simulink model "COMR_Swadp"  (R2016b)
settings: Solver=FixedStepDiscrete  StartTime=0.0  StopTime=10.0  FixedStep=0.02  RelTol=1e-3  EnableMultiTasking=on
undefined symbols (not defined in the file or in its folder): bin2dec, COMR_ahBattNrmCap_C, COMR_cntNvmReadErr_CW, COMR_ti638LinComErr_C, COMR_tiNvmReadErr_C
libraries: simulink x93, dspswit3 x2
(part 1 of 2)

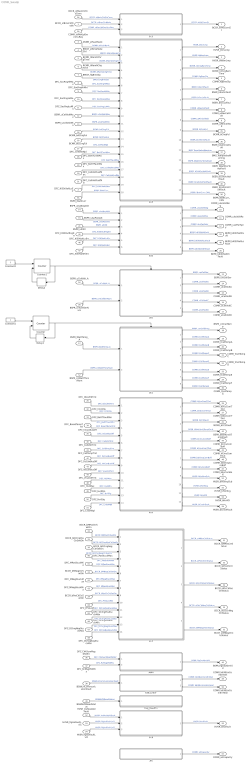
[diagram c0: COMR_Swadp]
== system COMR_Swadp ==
  BCCR_stBmsCtrMode : Inport
  DFC_Kl30cVoltLoErr : Inport  Port=2
  DSMR_stFaultRank : Inport  Port=3
  BMCR_stBmsModeCtrl : Inport  Port=4
  BCMR_tiRemDChrgTime : Inport  Port=5
  BCMR_tiRemAChgTime : Inport  Port=6
  BMCR_flgBmsSlp : Inport  Port=7
  DFC_SocRngHiMax : Inport  Port=8
  DFC_SocRngHiMin : Inport  Port=9
  DFC_SocRngLoMax : Inport  Port=10
  DFC_SocRngLoMin : Inport  Port=11
  BSPR_uCellVoltMax : Inport  Port=12
  BSPR_uCellVoltMin : Inport  Port=13
  BSPR_uIsoNegVolt : Inport  Port=14
  BSPR_uIsoPosVolt : Inport  Port=15
  BSPR_uCellVolt_A : Inport  Port=16
  BSPR_tBattTemp_A : Inport  Port=17
  BCMR_bAChrgFul : Inport  Port=18
  BCMR_bDChrgFul : Inport  Port=19
  DFC_Obc2E0Tmt : Inport  Port=20
  BSPR_uKl30 : Inport  Port=21
  BCCR_bMPosCtrSwtOn : Inport  Port=22
  BCCR_bMNegCtrSwtOn : Inport  Port=23
  BCCR_bPreChCtrSwtOn : Inport  Port=24
  BCCR_bDChrgPosCtrSwtOn : Inport  Port=25
  BCCR_bDChrgNegCtrSwtOn : Inport  Port=26
  DFC_CellVoltNpl : Inport  Port=27
  DFC_BattTCnstMax : Inport  Port=28
  DFC_BattTFaultMax : Inport  Port=29
  DFC_CellVoltFusfMax : Inport  Port=30
  DFC_CellVoltFusfMin : Inport  Port=31
  DFC_CC2Chk : Inport  Port=32
  DFC_BattTFaultMin : Inport  Port=33
  DFC_BoardTempTmt : Inport  Port=34
  DFC_InCanBusOff : Inport  Port=35
  DFC_ChkSumMsg050Err : Inport  Port=36
  DFC_RcMsg050Mis : Inport  Port=37
  BSWLinCommunicationFault : Inport  Port=38
  BSWNVMReadStatus : Inport  Port=39
  DFC_CellVoltTmt : Inport  Port=40
  DFC_CellTempTmt : Inport  Port=41
  DFC_DcCanBusOff : Inport  Port=42
  DFC_VeCanBusOff : Inport  Port=43
  DFC_Vcu2A3Tmt : Inport  Port=44
  DFC_Kl30OutRngErr : Inport  Port=45
  DFC_Kl30VoltLoErr : Inport  Port=46
  DFC_Kl30VoltHiErr : Inport  Port=47
  DFC_HvilMax : Inport  Port=48
  DFC_HvilMin : Inport  Port=49
  DFC_HvilSig : Inport  Port=50
  DFC_CrashNpl : Inport  Port=51
  HVSR_InsResValdFault : Inport  Port=52
  HVSR_flgIsoFaultLvl1 : Inport  Port=53
  HVSR_flgIsoFaultLvl2 : Inport  Port=54
  BSPR_iBattCurr : Inport  Port=55
  BCCR_stMainCtrDisConn : Inport  Port=56
  BSPR_cntBattTSnsrNum : Inport  Port=57
  BSPR_cntCellSerNum : Inport  Port=58
  COMR_stPwrUpDwnVcuReq : Inport  Port=59
  DFC_PosStuckMax : Inport  Port=60
  DFC_MPosStuckMin : Inport  Port=61
  DFC_MNegStuckMax : Inport  Port=62
  DFC_MNegStuckMin : Inport  Port=63
  DFC_PrStuckMin : Inport  Port=64
  DFC_DChrgPosStuckMax : Inport  Port=65
  DFC_DChrgPosStuckMin : Inport  Port=66
  DFC_DChrgNegStuckMax : Inport  Port=67
  DFC_DChrgNegStuckMin : Inport  Port=68
  2C2 : Subsystem
  2C8 : Subsystem
  2CE : Subsystem
  2CF : Subsystem
  3E0 : Subsystem
  3E1 : Subsystem
  615 : Subsystem
  616 : Subsystem
  638_LinErr : Subsystem
  ABM : Subsystem
  Ah : Subsystem
  Constant1 : Constant
  Constant2 : Constant
  Counter : dspswit3/Counter  Direction=Up  CountEvent=Non-zero sample  CounterSize=User defined  MaxCount=255  InitialCount=0  Output=Hit  HitValue=10  ResetInput=on  SamplesPerFrame=1  Ts=1  CntDtype=double  HitDtype=Logical
  Counter1 : dspswit3/Counter  Direction=Up  CountEvent=Non-zero sample  CounterSize=User defined  MaxCount=255  InitialCount=0  Output=Hit  HitValue=2  ResetInput=on  SamplesPerFrame=1  Ts=1  CntDtype=double  HitDtype=Logical
  Delay1 : Delay  DelayLength=1  InitialCondition=0
  Delay2 : Delay  DelayLength=1  InitialCondition=0
  Eep_ReadErr : Subsystem
  BCCR_stHVConnSt : Outport
  HVSR_bSrvLmp : Outport  Port=2
  HVSR_bWarnLmp : Outport  Port=3
  BCMR_tiChrgRemTime : Outport  Port=4
  COMR_flgBmsSlp : Outport  Port=5
  BSER_bSocHiFault : Outport  Port=6
  BSER_bSocLoFault : Outport  Port=7
  COMR_uMaxCellVolt : Outport  Port=8
  COMR_uMinCellVolt : Outport  Port=9
  COMR_uIsoVoltNeg : Outport  Port=10
  COMR_uIsoVoltPos : Outport  Port=11
  COMR_uLoPwrSply : Outport  Port=12
  BSPR_cntCellSer : Outport  Port=13
  COMR_uCellVoltA : Outport  Port=14
  COMR_uCellVoltB : Outport  Port=15
  COMR_uCellVoltC : Outport  Port=16
  COMR_uCellVoltD : Outport  Port=17
  BSPR_cntCellTemp : Outport  Port=18
  COMR_tCellTempA : Outport  Port=19
  COMR_tCellTempB : Outport  Port=20
  COMR_tCellTempC : Outport  Port=21
  COMR_tCellTempD : Outport  Port=22
  COMR_tCellTempE : Outport  Port=23
  COMR_tCellTempF : Outport  Port=24
  BCMR_bChrgFul : Outport  Port=25
  COMR_bVcuComTOut : Outport  Port=26
  COMR_bObcComTOut : Outport  Port=27
  BEPR_bKl30VoltHiFault : Outport  Port=28
  BEPR_bKl30VoltFault : Outport  Port=29
  COMR_tCellTempG : Outport  Port=30
  BCCR_stMPosCtrStatus : Outport  Port=31
  BCCR_stMNegChCtrStatus : Outport  Port=32
  BCCR_stPreChCtrStatus : Outport  Port=33
  BCCR_stDcChPosCtrStatus : Outport  Port=34
  BCCR_stDcChNegCtrStatus : Outport  Port=35
  BSER_bCellCnstFault : Outport  Port=36
  BMS_TempValueWarning : Outport  Port=37
  BSPR_bBattOvrTempFault : Outport  Port=38
  BSER_bCellOvrVoltFault : Outport  Port=39
  BSER_bCellUndrVoltFault : Outport  Port=40
  BCMR_bCC2Fault : Outport  Port=41
  BSPR_bBattUndrTempFault : Outport  Port=42
  COMR_bCmuComTOut : Outport  Port=43
  COMR_bCmuComBoff : Outport  Port=44
  BSPR_flgGwAbmVld : Outport  Port=45
  COMR_bDChrgComBoff : Outport  Port=46
  COMR_bEvComBoff : Outport  Port=47
  BEPR_bKl30VoltLoFault : Outport  Port=48
  COMR_b638LinComErrDet : Outport  Port=49
  COMR_b638LinComErrHeal : Outport  Port=50
  HVSR_bHvilInpScb : Outport  Port=51
  HVSR_bHvilScg : Outport  Port=52
  HVSR_bHvilOl : Outport  Port=53
  HVSR_bCrashFault : Outport  Port=54
  HVSR_bIsoFault : Outport  Port=55
  BSPR_iBattCurr_CAN : Outport  Port=56
  COMR_ahCapacity : Outport  Port=57
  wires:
  BSPR_uIsoPosVolt/1 -> 616/2(BSPR_uIsoPosVolt)  "BSPR_uIsoPosVolt"
  BSPR_uKl30/1 -> 616/3(BSPR_uKl30)  "BSPR_uKl30"
  DFC_SocRngHiMax/1 -> 2CE/6(DFC_SocRngHiMax)  "DFC_SocRngHiMax"
  DFC_SocRngHiMin/1 -> 2CE/7(DFC_SocRngHiMin)  "DFC_SocRngHiMin"
  DFC_SocRngLoMax/1 -> 2CE/8(DFC_SocRngLoMax)  "DFC_SocRngLoMax"
  DFC_SocRngLoMin/1 -> 2CE/9(DFC_SocRngLoMin)  "DFC_SocRngLoMin"
  BSPR_uCellVoltMax/1 -> 2CE/10(BSPR_uCellVoltMax)  "BSPR_uCellVoltMax"
  BSPR_uCellVoltMin/1 -> 2CE/11(BSPR_uCellVoltMin)  "BSPR_uCellVoltMin"
  2CE/8(COMR_uMinCellVolt) -> COMR_uMinCellVolt/1  "COMR_uMinCellVolt"
  2CE/7(COMR_uMaxCellVolt) -> COMR_uMaxCellVolt/1  "COMR_uMaxCellVolt"
  BSPR_uIsoNegVolt/1 -> 616/1(BSPR_uIsoNegVolt)  "BSPR_uIsoNegVolt"
  2CE/4(COMR_flgBmsSlp) -> COMR_flgBmsSlp/1  "COMR_flgBmsSlp"
  BMCR_flgBmsSlp/1 -> 2CE/5(BMCR_flgBmsSlp)  "BMCR_flgBmsSlp"
  2C2/1(BCCR_stHVConnSt) -> BCCR_stHVConnSt/1  "BCCR_stHVConnSt"
  616/2(COMR_uIsoVoltPos) -> COMR_uIsoVoltPos/1  "COMR_uIsoVoltPos"
  BMCR_stBmsModeCtrl/1 -> 2CE/2(BMCR_stBmsModeCtrl)  "BMCR_stBmsModeCtrl"
  2CE/3(BCMR_tiChrgRemTime) -> BCMR_tiChrgRemTime/1  "BCMR_tiChrgRemTime"
  2CE/2(HVSR_bWarnLmp) -> HVSR_bWarnLmp/1  "HVSR_bWarnLmp"
  616/3(COMR_uLoPwrSply) -> COMR_uLoPwrSply/1  "COMR_uLoPwrSply"
  DSMR_stFaultRank/1 -> 2CE/1(DSMR_stFaultRank)  "DSMR_stFaultRank"
  BCCR_stBmsCtrMode/1 -> 2C2/2(BCCR_stBmsCtrMode)  "BCCR_stBmsCtrMode"
  2CE/5(BSER_bSocHiFault) -> BSER_bSocHiFault/1  "BSER_bSocHiFault"
  2CE/6(BSER_bSocLoFault) -> BSER_bSocLoFault/1  "BSER_bSocLoFault"
  DFC_Kl30cVoltLoErr/1 -> 2CE/19(DFC_Kl30cVoltLoErr)  "DFC_Kl30cVoltLoErr"
  BCMR_tiRemDChrgTime/1 -> 2CE/3(BCMR_tiRemDChrgTime)  "BCMR_tiRemDChrgTime"
  2CE/1(HVSR_bSrvLmp) -> HVSR_bSrvLmp/1  "HVSR_bSrvLmp"
  616/1(COMR_uIsoVoltNeg) -> COMR_uIsoVoltNeg/1  "COMR_uIsoVoltNeg"
  BCMR_tiRemAChgTime/1 -> 2CE/4(BCMR_tiRemAChgTime)  "BCMR_tiRemAChgTime"
  BCMR_bDChrgFul/1 -> 2CE/13(BCMR_bDChrgFul)  "BCMR_bDChrgFul"
  BCMR_bAChrgFul/1 -> 2CE/12(BCMR_bAChrgFul)  "BCMR_bAChrgFul"
  2CE/9(BCMR_bChrgFul) -> BCMR_bChrgFul/1  "BCMR_bChrgFul"
  DFC_Obc2E0Tmt/1 -> 615/1(DFC_Obc2E0Tmt)  "DFC_Obc2E0Tmt"
  615/1(COMR_bVcuComTOut) -> COMR_bVcuComTOut/1  "COMR_bVcuComTOut"
  615/2(COMR_bObcComTOut) -> COMR_bObcComTOut/1  "COMR_bObcComTOut"
  616/4(BEPR_bKl30VoltFault) -> BEPR_bKl30VoltFault/1  "BEPR_bKl30VoltFault"
  616/6(BEPR_bKl30VoltHiFault) -> BEPR_bKl30VoltHiFault/1  "BEPR_bKl30VoltHiFault"
  BSPR_uCellVolt_A/1 -> 3E0/1(BSPR_uCellVolt_A)  "BSPR_uCellVolt_A"
  3E0/1(BSPR_cntCellSer) -> BSPR_cntCellSer/1  "BSPR_cntCellSer"
  3E0/2(COMR_uCellVoltA) -> COMR_uCellVoltA/1  "COMR_uCellVoltA"
  3E0/3(COMR_uCellVoltB) -> COMR_uCellVoltB/1  "COMR_uCellVoltB"
  3E0/4(COMR_uCellVoltC) -> COMR_uCellVoltC/1  "COMR_uCellVoltC"
  3E0/5(COMR_uCellVoltD) -> COMR_uCellVoltD/1  "COMR_uCellVoltD"
  BSPR_tBattTemp_A/1 -> 3E1/1(BSPR_tBattTemp_A)  "BSPR_tBattTemp_A"
  3E1/1(BSPR_cntCellTemp) -> BSPR_cntCellTemp/1  "BSPR_cntCellTemp"
  3E1/2(COMR_tCellTempA) -> COMR_tCellTempA/1  "COMR_tCellTempA"
  3E1/3(COMR_tCellTempB) -> COMR_tCellTempB/1  "COMR_tCellTempB"
  3E1/4(COMR_tCellTempC) -> COMR_tCellTempC/1  "COMR_tCellTempC"
  3E1/5(COMR_tCellTempD) -> COMR_tCellTempD/1  "COMR_tCellTempD"
  3E1/6(COMR_tCellTempE) -> COMR_tCellTempE/1  "COMR_tCellTempE"
  3E1/7(COMR_tCellTempF) -> COMR_tCellTempF/1  "COMR_tCellTempF"
  Constant1/1 -> Counter/1
  Delay1/1 -> Counter/2
  Counter/1 -> 3E1/Enable, Delay1/1
  Constant2/1 -> Counter1/1
  Delay2/1 -> Counter1/2
  Counter1/1 -> 3E0/Enable, Delay2/1
  3E1/8(COMR_tCellTempG) -> COMR_tCellTempG/1  "COMR_tCellTempG"
  BCCR_bMPosCtrSwtOn/1 -> 2CF/1(BCCR_bMPosCtrSwtOn)  "BCCR_bMPosCtrSwtOn"
  BCCR_bMNegCtrSwtOn/1 -> 2CF/6(BCCR_bMNegCtrSwtOn)  "BCCR_bMNegCtrSwtOn"
  BCCR_bPreChCtrSwtOn/1 -> 2CF/9(BCCR_bPreChCtrSwtOn)  "BCCR_bPreChCtrSwtOn"
  BCCR_bDChrgPosCtrSwtOn/1 -> 2CF/2(BCCR_bDChrgPosCtrSwtOn)  "BCCR_bDChrgPosCtrSwtOn"
  BCCR_bDChrgNegCtrSwtOn/1 -> 2CF/3(BCCR_bDChrgNegCtrSwtOn)  "BCCR_bDChrgNegCtrSwtOn"
  2CF/1(BCCR_stMPosCtrStatus) -> BCCR_stMPosCtrStatus/1  "BCCR_stMPosCtrStatus"
  2CF/5(BCCR_stMNegChCtrStatus) -> BCCR_stMNegChCtrStatus/1  "BCCR_stMNegChCtrStatus"
  2CF/2(BCCR_stPreChCtrStatus) -> BCCR_stPreChCtrStatus/1  "BCCR_stPreChCtrStatus"
  2CF/3(BCCR_stDcChPosCtrStatus) -> BCCR_stDcChPosCtrStatus/1  "BCCR_stDcChPosCtrStatus"
  2CF/4(BCCR_stDcChNegCtrStatus) -> BCCR_stDcChNegCtrStatus/1  "BCCR_stDcChNegCtrStatus"
  2CE/10(BSER_bCellCnstFault) -> BSER_bCellCnstFault/1  "BSER_bCellCnstFault"
  2CE/11(BMS_TempValueWarning) -> BMS_TempValueWarning/1  "BMS_TempValueWarning"
  2CE/12(BSPR_bBattOvrTempFault) -> BSPR_bBattOvrTempFault/1  "BSPR_bBattOvrTempFault"
  2CE/13(BSER_bCellOvrVoltFault) -> BSER_bCellOvrVoltFault/1  "BSER_bCellOvrVoltFault"
  2CE/14(BSER_bCellUndrVoltFault) -> BSER_bCellUndrVoltFault/1  "BSER_bCellUndrVoltFault"
  DFC_CellVoltNpl/1 -> 2CE/14(DFC_CellVoltNpl)  "DFC_CellVoltNpl"
  DFC_BattTCnstMax/1 -> 2CE/15(DFC_BattTCnstMax)  "DFC_BattTCnstMax"
  DFC_BattTFaultMax/1 -> 2CE/16(DFC_BattTFaultMax)  "DFC_BattTFaultMax"
  DFC_CellVoltFusfMax/1 -> 2CE/17(DFC_CellVoltFusfMax)  "DFC_CellVoltFusfMax"
  DFC_CellVoltFusfMin/1 -> 2CE/18(DFC_CellVoltFusfMin)  "DFC_CellVoltFusfMin"
  615/4(BSPR_bBattUndrTempFault) -> BSPR_bBattUndrTempFault/1  "BSPR_bBattUndrTempFault"
  615/3(BCMR_bCC2Fault) -> BCMR_bCC2Fault/1  "BCMR_bCC2Fault"
  DFC_BattTFaultMin/1 -> 615/3(DFC_BattTFaultMin)  "DFC_BattTFaultMin"
  DFC_CC2Chk/1 -> 615/2(DFC_CC2Chk)  "DFC_CC2Chk"
  DFC_BoardTempTmt/1 -> 615/4(DFC_BoardTempTmt)  "DFC_BoardTempTmt"
  DFC_InCanBusOff/1 -> 615/5(DFC_InCanBusOff)  "DFC_InCanBusOff"
  615/6(COMR_bCmuComTOut) -> COMR_bCmuComTOut/1  "COMR_bCmuComTOut"
  615/5(COMR_bCmuComBoff) -> COMR_bCmuComBoff/1  "COMR_bCmuComBoff"
  DFC_ChkSumMsg050Err/1 -> ABM/1(DFC_ChkSumMsg050Err)  "DFC_ChkSumMsg050Err"
  DFC_RcMsg050Mis/1 -> ABM/2(DFC_RcMsg050Mis)  "DFC_RcMsg050Mis"
  ABM/1(BSPR_flgGwAbmVld) -> BSPR_flgGwAbmVld/1  "BSPR_flgGwAbmVld"
  BSWLinCommunicationFault/1 -> 638_LinErr/1(BSWLinCommunicationFault)  "BSWLinCommunicationFault"
  BSWNVMReadStatus/1 -> Eep_ReadErr/1(BSWNVMReadStatus)  "BSWNVMReadStatus"
  DFC_CellVoltTmt/1 -> 615/6(DFC_CellVoltTmt)  "DFC_CellVoltTmt"
  DFC_CellTempTmt/1 -> 615/7(DFC_CellTempTmt)  "DFC_CellTempTmt"
  615/7(COMR_bDChrgComBoff) -> COMR_bDChrgComBoff/1  "COMR_bDChrgComBoff"
  615/8(COMR_bEvComBoff) -> COMR_bEvComBoff/1  "COMR_bEvComBoff"
  DFC_DcCanBusOff/1 -> 615/8(DFC_DcCanBusOff)  "DFC_DcCanBusOff"
  DFC_VeCanBusOff/1 -> 615/9(DFC_VeCanBusOff)  "DFC_VeCanBusOff"
  DFC_Vcu2A3Tmt/1 -> 615/10(DFC_Vcu2A3Tmt)  "DFC_Vcu2A3Tmt"
  616/5(BEPR_bKl30VoltLoFault) -> BEPR_bKl30VoltLoFault/1  "BEPR_bKl30VoltLoFault"
  DFC_Kl30OutRngErr/1 -> 616/4(DFC_Kl30OutRngErr)  "DFC_Kl30OutRngErr"
  DFC_Kl30VoltLoErr/1 -> 616/5(DFC_Kl30VoltLoErr)  "DFC_Kl30VoltLoErr"
  DFC_Kl30VoltHiErr/1 -> 616/6(DFC_Kl30VoltHiErr)  "DFC_Kl30VoltHiErr"
  638_LinErr/1(COMR_b638LinComErrDet) -> COMR_b638LinComErrDet/1  "COMR_b638LinComErrDet"
  638_LinErr/2(COMR_b638LinComErrHeal) -> COMR_b638LinComErrHeal/1  "COMR_b638LinComErrHeal"
  615/10(HVSR_bHvilScg) -> HVSR_bHvilScg/1  "HVSR_bHvilScg"
  615/9(HVSR_bHvilInpScb) -> HVSR_bHvilInpScb/1  "HVSR_bHvilInpScb"
  615/11(HVSR_bHvilOl) -> HVSR_bHvilOl/1  "HVSR_bHvilOl"
  615/12(HVSR_bCrashFault) -> HVSR_bCrashFault/1  "HVSR_bCrashFault"
  DFC_HvilMax/1 -> 615/11(DFC_HvilMax)  "DFC_HvilMax"
  DFC_HvilMin/1 -> 615/12(DFC_HvilMin)  "DFC_HvilMin"
  DFC_HvilSig/1 -> 615/13(DFC_HvilSig)  "DFC_HvilSig"
  DFC_CrashNpl/1 -> 615/14(DFC_CrashNpl)  "DFC_CrashNpl"
  HVSR_InsResValdFault/1 -> 2C8/1(HVSR_InsResValdFault)  "HVSR_InsResValdFault"
  HVSR_flgIsoFaultLvl1/1 -> 2C8/2(HVSR_flgIsoFaultLvl1)  "HVSR_flgIsoFaultLvl1"
  HVSR_flgIsoFaultLvl2/1 -> 2C8/3(HVSR_flgIsoFaultLvl2)  "HVSR_flgIsoFaultLvl2"
  2C8/1(HVSR_bIsoFault) -> HVSR_bIsoFault/1  "HVSR_bIsoFault"
  BSPR_iBattCurr/1 -> 2CE/20(BSPR_iBattCurr)  "BSPR_iBattCurr"
  2CE/15(BSPR_iBattCurr_CAN) -> BSPR_iBattCurr_CAN/1  "BSPR_iBattCurr_CAN"
  BCCR_stMainCtrDisConn/1 -> 2C2/1(BCCR_stMainCtrDisConn)  "BCCR_stMainCtrDisConn"
  BSPR_cntBattTSnsrNum/1 -> 3E1/2(BSPR_cntBattTSnsrNum)  "BSPR_cntBattTSnsrNum"
  BSPR_cntCellSerNum/1 -> 3E0/2(BSPR_cntCellSerNum)  "BSPR_cntCellSerNum"
  COMR_stPwrUpDwnVcuReq/1 -> 2C2/3(COMR_stPwrUpDwnVcuReq)  "COMR_stPwrUpDwnVcuReq"
  DFC_PosStuckMax/1 -> 2CF/4(DFC_PosStuckMax)  "DFC_PosStuckMax"
  DFC_MPosStuckMin/1 -> 2CF/5(DFC_MPosStuckMin)  "DFC_MPosStuckMin"
  DFC_MNegStuckMax/1 -> 2CF/7(DFC_MNegStuckMax)  "DFC_MNegStuckMax"
  DFC_MNegStuckMin/1 -> 2CF/8(DFC_MNegStuckMin)  "DFC_MNegStuckMin"
  DFC_PrStuckMin/1 -> 2CF/10(DFC_PrStuckMin)  "DFC_PrStuckMin"
  DFC_DChrgPosStuckMax/1 -> 2CF/11(DFC_DChrgPosStuckMax)  "DFC_DChrgPosStuckMax"
  DFC_DChrgPosStuckMin/1 -> 2CF/12(DFC_DChrgPosStuckMin)  "DFC_DChrgPosStuckMin"
  DFC_DChrgNegStuckMax/1 -> 2CF/13(DFC_DChrgNegStuckMax)  "DFC_DChrgNegStuckMax"
  DFC_DChrgNegStuckMin/1 -> 2CF/14(DFC_DChrgNegStuckMin)  "DFC_DChrgNegStuckMin"
  Ah/1(COMR_ahCapacity) -> COMR_ahCapacity/1  "COMR_ahCapacity"

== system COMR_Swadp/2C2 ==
  BCCR_stMainCtrDisConn : Inport
  BCCR_stBmsCtrMode : Inport  Port=2  OutDataTypeStr=uint8
  COMR_stPwrUpDwnVcuReq : Inport  Port=3
  HvCnttCalc : Stateflow chart  TreatAsAtomicUnit=on
  BCCR_stHVConnSt : Outport
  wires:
  HvCnttCalc/1(BCCR_stHVConnSt) -> BCCR_stHVConnSt/1
  BCCR_stBmsCtrMode/1 -> HvCnttCalc/1(BCCR_stBmsCtrMode)
  BCCR_stMainCtrDisConn/1 -> HvCnttCalc/3(BCCR_stMainCtrDisConn)
  COMR_stPwrUpDwnVcuReq/1 -> HvCnttCalc/2(COMR_stPwrUpDwnVcuReq)

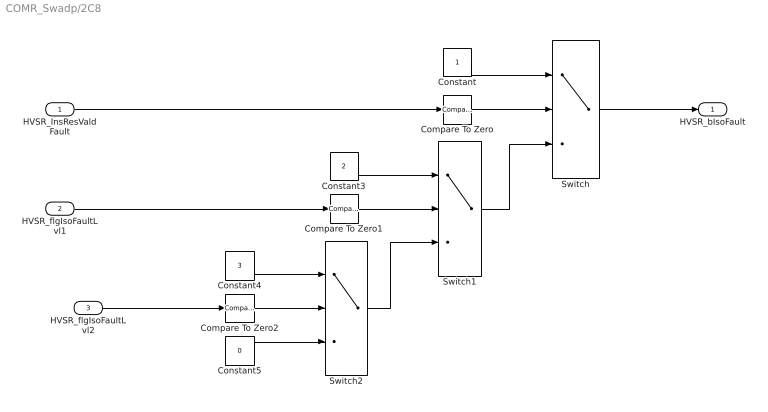
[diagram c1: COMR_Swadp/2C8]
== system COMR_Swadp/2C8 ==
  HVSR_InsResValdFault : Inport
  HVSR_flgIsoFaultLvl1 : Inport  Port=2
  HVSR_flgIsoFaultLvl2 : Inport  Port=3
  Compare To Zero : simulink/Logic and Bit Operations/Compare To Zero  relop=~=  OutDataTypeStr=boolean
  Compare To Zero1 : simulink/Logic and Bit Operations/Compare To Zero  relop=~=  OutDataTypeStr=boolean
  Compare To Zero2 : simulink/Logic and Bit Operations/Compare To Zero  relop=~=  OutDataTypeStr=boolean
  Constant : Constant  OutDataTypeStr=uint8
  Constant3 : Constant  Value=2  OutDataTypeStr=uint8
  Constant4 : Constant  Value=3  OutDataTypeStr=uint8
  Constant5 : Constant  Value=0  OutDataTypeStr=uint8
  Switch : Switch  Criteria=u2 > Threshold
  Switch1 : Switch  Criteria=u2 > Threshold
  Switch2 : Switch  Criteria=u2 > Threshold
  HVSR_bIsoFault : Outport
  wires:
  Switch/1 -> HVSR_bIsoFault/1
  HVSR_flgIsoFaultLvl1/1 -> Compare To Zero1/1
  Switch1/1 -> Switch/3
  Constant5/1 -> Switch2/3
  Switch2/1 -> Switch1/3
  Constant4/1 -> Switch2/1
  Compare To Zero1/1 -> Switch1/2
  Constant/1 -> Switch/1
  Constant3/1 -> Switch1/1
  Compare To Zero2/1 -> Switch2/2
  HVSR_flgIsoFaultLvl2/1 -> Compare To Zero2/1
  HVSR_InsResValdFault/1 -> Compare To Zero/1
  Compare To Zero/1 -> Switch/2

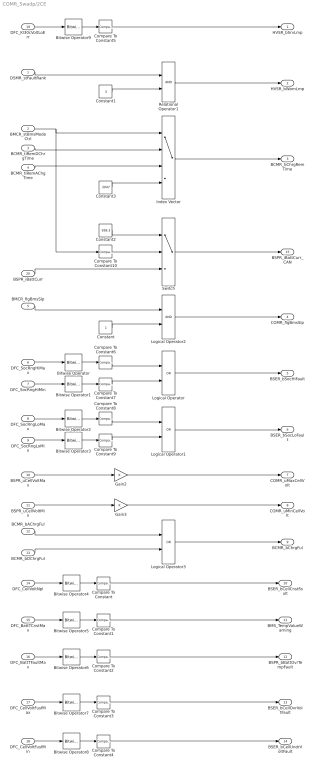
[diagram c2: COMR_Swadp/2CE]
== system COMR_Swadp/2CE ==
  DSMR_stFaultRank : Inport
  BMCR_stBmsModeCtrl : Inport  Port=2
  BCMR_tiRemDChrgTime : Inport  Port=3
  BCMR_tiRemAChgTime : Inport  Port=4
  BMCR_flgBmsSlp : Inport  Port=5
  DFC_SocRngHiMax : Inport  Port=6
  DFC_SocRngHiMin : Inport  Port=7
  DFC_SocRngLoMax : Inport  Port=8
  DFC_SocRngLoMin : Inport  Port=9
  BSPR_uCellVoltMax : Inport  Port=10
  BSPR_uCellVoltMin : Inport  Port=11
  BCMR_bAChrgFul : Inport  Port=12
  BCMR_bDChrgFul : Inport  Port=13
  DFC_CellVoltNpl : Inport  Port=14
  DFC_BattTCnstMax : Inport  Port=15
  DFC_BattTFaultMax : Inport  Port=16
  DFC_CellVoltFusfMax : Inport  Port=17
  DFC_CellVoltFusfMin : Inport  Port=18
  DFC_Kl30cVoltLoErr : Inport  Port=19
  BSPR_iBattCurr : Inport  Port=20
  Bitwise Operator{,1..9} (10 alike) : simulink/Logic and Bit Operations/Bitwise Operator  logicop=AND  UseBitMask=on  BitMask=bin2dec('00011000')  BitMaskRealWorld=Stored Integer
  Compare To Constant{,1..9} (10 alike) : simulink/Logic and Bit Operations/Compare To Constant  relop===  const=24  OutDataTypeStr=boolean
  Compare To Constant10 : simulink/Logic and Bit Operations/Compare To Constant  relop===  const=11  OutDataTypeStr=boolean
  Constant : Constant  OutDataTypeStr=boolean
  Constant1 : Constant  Value=3  OutDataTypeStr=uint8
  Constant2 : Constant  Value=938.3  OutDataTypeStr=single
  Constant3 : Constant  Value=2047  OutDataTypeStr=single
  Gain2 : Gain
  Gain3 : Gain
  Index Vector : MultiPortSwitch  DataPortOrder=Specify indices  Inputs=1  DataPortIndices={5,6}  DataPortForDefault=Additional data port  DiagnosticForDefault=None  OutDataTypeStr=single
  Logical Operator : Logic  Operator=OR  AllPortsSameDT=off  OutDataTypeStr=boolean
  Logical Operator1 : Logic  Operator=OR  AllPortsSameDT=off  OutDataTypeStr=boolean
  Logical Operator2 : Logic  AllPortsSameDT=off  OutDataTypeStr=boolean
  Logical Operator3 : Logic  Operator=OR  AllPortsSameDT=off  OutDataTypeStr=boolean
  Relational Operator1 : RelationalOperator  OutDataTypeStr=boolean  RndMeth=Simplest
  Switch : Switch  Criteria=u2 > Threshold
  HVSR_bSrvLmp : Outport
  HVSR_bWarnLmp : Outport  Port=2
  BCMR_tiChrgRemTime : Outport  Port=3
  COMR_flgBmsSlp : Outport  Port=4  OutDataTypeStr=boolean
  BSER_bSocHiFault : Outport  Port=5  OutDataTypeStr=boolean
  BSER_bSocLoFault : Outport  Port=6  OutDataTypeStr=boolean
  COMR_uMaxCellVolt : Outport  Port=7
  COMR_uMinCellVolt : Outport  Port=8
  BCMR_bChrgFul : Outport  Port=9
  BSER_bCellCnstFault : Outport  Port=10
  BMS_TempValueWarning : Outport  Port=11
  BSPR_bBattOvrTempFault : Outport  Port=12
  BSER_bCellOvrVoltFault : Outport  Port=13
  BSER_bCellUndrVoltFault : Outport  Port=14
  BSPR_iBattCurr_CAN : Outport  Port=15
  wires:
  Index Vector/1 -> BCMR_tiChrgRemTime/1
  BCMR_tiRemDChrgTime/1 -> Index Vector/2
  BMCR_stBmsModeCtrl/1 -> Compare To Constant10/1, Index Vector/1
  BCMR_tiRemAChgTime/1 -> Index Vector/3
  Relational Operator1/1 -> HVSR_bWarnLmp/1
  DSMR_stFaultRank/1 -> Relational Operator1/1
  Constant1/1 -> Relational Operator1/2
  DFC_SocRngHiMax/1 -> Bitwise Operator/1
  DFC_SocRngHiMin/1 -> Bitwise Operator1/1
  Bitwise Operator/1 -> Compare To Constant6/1
  Bitwise Operator1/1 -> Compare To Constant7/1
  Logical Operator/1 -> BSER_bSocHiFault/1
  DFC_SocRngLoMax/1 -> Bitwise Operator2/1
  DFC_SocRngLoMin/1 -> Bitwise Operator3/1
  Bitwise Operator2/1 -> Compare To Constant8/1
  Bitwise Operator3/1 -> Compare To Constant9/1
  Logical Operator1/1 -> BSER_bSocLoFault/1
  BSPR_uCellVoltMax/1 -> Gain2/1
  BSPR_uCellVoltMin/1 -> Gain3/1
  Gain2/1 -> COMR_uMaxCellVolt/1
  Gain3/1 -> COMR_uMinCellVolt/1
  BMCR_flgBmsSlp/1 -> Logical Operator2/1
  Constant/1 -> Logical Operator2/2
  Logical Operator2/1 -> COMR_flgBmsSlp/1
  Constant3/1 -> Index Vector/4
  Logical Operator3/1 -> BCMR_bChrgFul/1
  BCMR_bAChrgFul/1 -> Logical Operator3/1
  BCMR_bDChrgFul/1 -> Logical Operator3/2
  Bitwise Operator4/1 -> Compare To Constant/1
  DFC_CellVoltNpl/1 -> Bitwise Operator4/1
  DFC_BattTCnstMax/1 -> Bitwise Operator5/1
  Bitwise Operator5/1 -> Compare To Constant1/1
  DFC_BattTFaultMax/1 -> Bitwise Operator6/1
  Bitwise Operator6/1 -> Compare To Constant2/1
  DFC_CellVoltFusfMax/1 -> Bitwise Operator7/1
  Bitwise Operator7/1 -> Compare To Constant3/1
  DFC_CellVoltFusfMin/1 -> Bitwise Operator8/1
  Bitwise Operator8/1 -> Compare To Constant4/1
  Compare To Constant/1 -> BSER_bCellCnstFault/1
  Compare To Constant1/1 -> BMS_TempValueWarning/1
  Compare To Constant2/1 -> BSPR_bBattOvrTempFault/1
  Compare To Constant3/1 -> BSER_bCellOvrVoltFault/1
  Compare To Constant4/1 -> BSER_bCellUndrVoltFault/1
  DFC_Kl30cVoltLoErr/1 -> Bitwise Operator9/1
  Bitwise Operator9/1 -> Compare To Constant5/1
  Compare To Constant5/1 -> HVSR_bSrvLmp/1
  Compare To Constant6/1 -> Logical Operator/1
  Compare To Constant7/1 -> Logical Operator/2
  Compare To Constant8/1 -> Logical Operator1/1
  Compare To Constant9/1 -> Logical Operator1/2
  Compare To Constant10/1 -> Switch/2
  Constant2/1 -> Switch/1
  BSPR_iBattCurr/1 -> Switch/3
  Switch/1 -> BSPR_iBattCurr_CAN/1

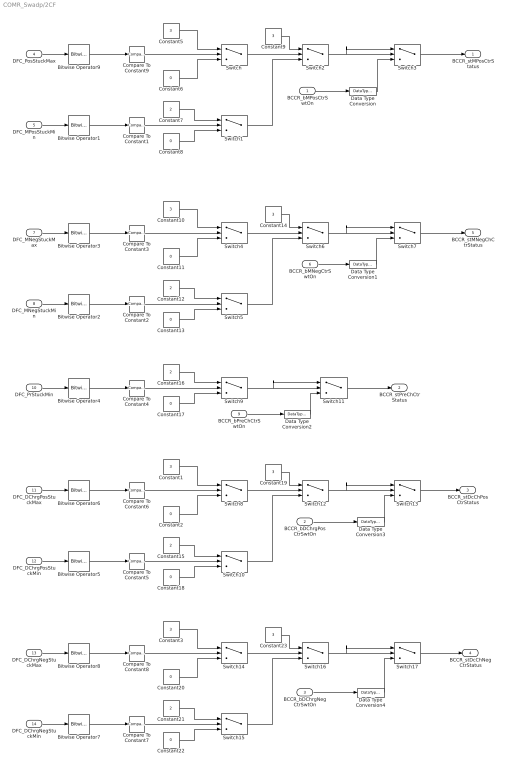
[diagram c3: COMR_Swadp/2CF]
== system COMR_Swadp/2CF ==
  BCCR_bMPosCtrSwtOn : Inport
  BCCR_bDChrgPosCtrSwtOn : Inport  Port=2
  BCCR_bDChrgNegCtrSwtOn : Inport  Port=3
  DFC_PosStuckMax : Inport  Port=4
  DFC_MPosStuckMin : Inport  Port=5
  BCCR_bMNegCtrSwtOn : Inport  Port=6
  DFC_MNegStuckMax : Inport  Port=7
  DFC_MNegStuckMin : Inport  Port=8
  BCCR_bPreChCtrSwtOn : Inport  Port=9
  DFC_PrStuckMin : Inport  Port=10
  DFC_DChrgPosStuckMax : Inport  Port=11
  DFC_DChrgPosStuckMin : Inport  Port=12
  DFC_DChrgNegStuckMax : Inport  Port=13
  DFC_DChrgNegStuckMin : Inport  Port=14
  Bitwise Operator{1..9} (9 alike) : simulink/Logic and Bit Operations/Bitwise Operator  logicop=AND  UseBitMask=on  BitMask=bin2dec('00011000')  BitMaskRealWorld=Stored Integer
  Compare To Constant{1..9} (9 alike) : simulink/Logic and Bit Operations/Compare To Constant  relop===  const=24  OutDataTypeStr=boolean
  Constant{1,3,5,9..10,14,19,23} (8 alike) : Constant  Value=3  OutDataTypeStr=uint8
  Constant{2,6,8,11,13,17..18,20,22} (9 alike) : Constant  Value=0  OutDataTypeStr=uint8
  Constant{7,12,15..16,21} (5 alike) : Constant  Value=2  OutDataTypeStr=uint8
  Data Type Conversion{,1..4} (5 alike) : DataTypeConversion  OutDataTypeStr=uint8
  Switch{,1..17} (18 alike) : Switch  Criteria=u2 ~= 0
  BCCR_stMPosCtrStatus : Outport
  BCCR_stPreChCtrStatus : Outport  Port=2
  BCCR_stDcChPosCtrStatus : Outport  Port=3
  BCCR_stDcChNegCtrStatus : Outport  Port=4
  BCCR_stMNegChCtrStatus : Outport  Port=5
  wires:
  DFC_PosStuckMax/1 -> Bitwise Operator9/1
  Bitwise Operator9/1 -> Compare To Constant9/1
  Compare To Constant9/1 -> Switch/2
  Constant5/1 -> Switch/1
  Constant6/1 -> Switch/3
  Bitwise Operator1/1 -> Compare To Constant1/1
  Compare To Constant1/1 -> Switch1/2
  DFC_MPosStuckMin/1 -> Bitwise Operator1/1
  Constant7/1 -> Switch1/1
  Constant8/1 -> Switch1/3
  Switch/1 -> Switch2/2
  Constant9/1 -> Switch2/1
  Switch1/1 -> Switch2/3
  Switch2/1 -> Switch3/1, Switch3/2
  BCCR_bMPosCtrSwtOn/1 -> Data Type Conversion/1
  Switch3/1 -> BCCR_stMPosCtrStatus/1
  DFC_MNegStuckMax/1 -> Bitwise Operator3/1
  Bitwise Operator3/1 -> Compare To Constant3/1
  Compare To Constant3/1 -> Switch4/2
  Constant10/1 -> Switch4/1
  Constant11/1 -> Switch4/3
  Bitwise Operator2/1 -> Compare To Constant2/1
  Compare To Constant2/1 -> Switch5/2
  DFC_MNegStuckMin/1 -> Bitwise Operator2/1
  Constant12/1 -> Switch5/1
  Constant13/1 -> Switch5/3
  Switch4/1 -> Switch6/2
  Constant14/1 -> Switch6/1
  Switch5/1 -> Switch6/3
  Switch6/1 -> Switch7/1, Switch7/2
  BCCR_bMNegCtrSwtOn/1 -> Data Type Conversion1/1
  Switch7/1 -> BCCR_stMNegChCtrStatus/1
  Bitwise Operator4/1 -> Compare To Constant4/1
  Compare To Constant4/1 -> Switch9/2
  DFC_PrStuckMin/1 -> Bitwise Operator4/1
  Constant16/1 -> Switch9/1
  Constant17/1 -> Switch9/3
  Switch9/1 -> Switch11/1, Switch11/2
  BCCR_bPreChCtrSwtOn/1 -> Data Type Conversion2/1
  Switch11/1 -> BCCR_stPreChCtrStatus/1
  DFC_DChrgPosStuckMax/1 -> Bitwise Operator6/1
  Bitwise Operator6/1 -> Compare To Constant6/1
  Compare To Constant6/1 -> Switch8/2
  Constant1/1 -> Switch8/1
  Constant2/1 -> Switch8/3
  Bitwise Operator5/1 -> Compare To Constant5/1
  Compare To Constant5/1 -> Switch10/2
  DFC_DChrgPosStuckMin/1 -> Bitwise Operator5/1
  Constant15/1 -> Switch10/1
  Constant18/1 -> Switch10/3
  Switch8/1 -> Switch12/2
  Constant19/1 -> Switch12/1
  Switch10/1 -> Switch12/3
  Switch12/1 -> Switch13/1, Switch13/2
  BCCR_bDChrgPosCtrSwtOn/1 -> Data Type Conversion3/1
  Switch13/1 -> BCCR_stDcChPosCtrStatus/1
  DFC_DChrgNegStuckMax/1 -> Bitwise Operator8/1
  Bitwise Operator8/1 -> Compare To Constant8/1
  Compare To Constant8/1 -> Switch14/2
  Constant3/1 -> Switch14/1
  Constant20/1 -> Switch14/3
  Bitwise Operator7/1 -> Compare To Constant7/1
  Compare To Constant7/1 -> Switch15/2
  DFC_DChrgNegStuckMin/1 -> Bitwise Operator7/1
  Constant21/1 -> Switch15/1
  Constant22/1 -> Switch15/3
  Switch14/1 -> Switch16/2
  Constant23/1 -> Switch16/1
  Switch15/1 -> Switch16/3
  Switch16/1 -> Switch17/1, Switch17/2
  BCCR_bDChrgNegCtrSwtOn/1 -> Data Type Conversion4/1
  Switch17/1 -> BCCR_stDcChNegCtrStatus/1
  Data Type Conversion/1 -> Switch3/3
  Data Type Conversion1/1 -> Switch7/3
  Data Type Conversion2/1 -> Switch11/3
  Data Type Conversion3/1 -> Switch13/3
  Data Type Conversion4/1 -> Switch17/3

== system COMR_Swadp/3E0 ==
  BSPR_uCellVolt_A : Inport
  BSPR_cntCellSerNum : Inport  Port=2
  Enable : EnablePort
  3E0 : Stateflow chart  TreatAsAtomicUnit=on
  BSPR_cntCellSer : Outport
  COMR_uCellVoltA : Outport  Port=2
  COMR_uCellVoltB : Outport  Port=3
  COMR_uCellVoltC : Outport  Port=4
  COMR_uCellVoltD : Outport  Port=5
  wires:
  3E0/2(COMR_uCellVoltA) -> COMR_uCellVoltA/1
  3E0/4(COMR_uCellVoltC) -> COMR_uCellVoltC/1
  3E0/3(COMR_uCellVoltB) -> COMR_uCellVoltB/1
  BSPR_uCellVolt_A/1 -> 3E0/1(BSPR_uCellVolt_A)
  3E0/1(BSPR_cntCellSer) -> BSPR_cntCellSer/1
  3E0/5(COMR_uCellVoltD) -> COMR_uCellVoltD/1
  BSPR_cntCellSerNum/1 -> 3E0/2(BSPR_cntCellSerNum)

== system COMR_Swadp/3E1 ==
  BSPR_tBattTemp_A : Inport
  BSPR_cntBattTSnsrNum : Inport  Port=2
  Enable : EnablePort
  3E1 : Stateflow chart  TreatAsAtomicUnit=on
  BSPR_cntCellTemp : Outport
  COMR_tCellTempA : Outport  Port=2
  COMR_tCellTempB : Outport  Port=3
  COMR_tCellTempC : Outport  Port=4
  COMR_tCellTempD : Outport  Port=5
  COMR_tCellTempE : Outport  Port=6
  COMR_tCellTempF : Outport  Port=7
  COMR_tCellTempG : Outport  Port=8
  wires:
  3E1/1(BSPR_cntCellTemp) -> BSPR_cntCellTemp/1
  3E1/4(COMR_tCellTempC) -> COMR_tCellTempC/1
  BSPR_tBattTemp_A/1 -> 3E1/1(BSPR_tBattTemp_A)
  3E1/7(COMR_tCellTempF) -> COMR_tCellTempF/1
  3E1/6(COMR_tCellTempE) -> COMR_tCellTempE/1
  3E1/2(COMR_tCellTempA) -> COMR_tCellTempA/1
  3E1/3(COMR_tCellTempB) -> COMR_tCellTempB/1
  3E1/5(COMR_tCellTempD) -> COMR_tCellTempD/1
  3E1/8(COMR_tCellTempG) -> COMR_tCellTempG/1
  BSPR_cntBattTSnsrNum/1 -> 3E1/2(BSPR_cntBattTSnsrNum)

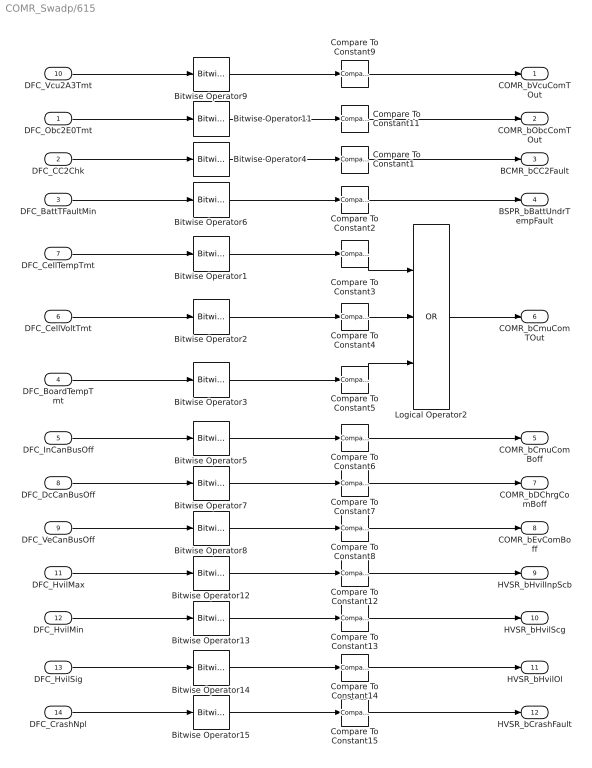
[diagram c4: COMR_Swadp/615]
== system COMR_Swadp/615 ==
  DFC_Obc2E0Tmt : Inport
  DFC_CC2Chk : Inport  Port=2
  DFC_BattTFaultMin : Inport  Port=3
  DFC_BoardTempTmt : Inport  Port=4
  DFC_InCanBusOff : Inport  Port=5
  DFC_CellVoltTmt : Inport  Port=6
  DFC_CellTempTmt : Inport  Port=7
  DFC_DcCanBusOff : Inport  Port=8
  DFC_VeCanBusOff : Inport  Port=9
  DFC_Vcu2A3Tmt : Inport  Port=10
  DFC_HvilMax : Inport  Port=11
  DFC_HvilMin : Inport  Port=12
  DFC_HvilSig : Inport  Port=13
  DFC_CrashNpl : Inport  Port=14
  Bitwise Operator{1..9,11..15} (14 alike) : simulink/Logic and Bit Operations/Bitwise Operator  logicop=AND  UseBitMask=on  BitMask=bin2dec('00011000')  BitMaskRealWorld=Stored Integer
  Compare To Constant{1..9,11..15} (14 alike) : simulink/Logic and Bit Operations/Compare To Constant  relop===  const=24  OutDataTypeStr=boolean
  Logical Operator2 : Logic  Operator=OR  Inputs=3  AllPortsSameDT=off  OutDataTypeStr=boolean
  COMR_bVcuComTOut : Outport
  COMR_bObcComTOut : Outport  Port=2
  BCMR_bCC2Fault : Outport  Port=3
  BSPR_bBattUndrTempFault : Outport  Port=4
  COMR_bCmuComBoff : Outport  Port=5
  COMR_bCmuComTOut : Outport  Port=6
  COMR_bDChrgComBoff : Outport  Port=7
  COMR_bEvComBoff : Outport  Port=8
  HVSR_bHvilInpScb : Outport  Port=9
  HVSR_bHvilScg : Outport  Port=10
  HVSR_bHvilOl : Outport  Port=11
  HVSR_bCrashFault : Outport  Port=12
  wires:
  DFC_Vcu2A3Tmt/1 -> Bitwise Operator9/1
  Compare To Constant11/1 -> COMR_bObcComTOut/1
  Bitwise Operator4/1 -> Compare To Constant1/1
  DFC_CC2Chk/1 -> Bitwise Operator4/1
  DFC_BattTFaultMin/1 -> Bitwise Operator6/1
  Bitwise Operator6/1 -> Compare To Constant2/1
  Compare To Constant1/1 -> BCMR_bCC2Fault/1
  Compare To Constant2/1 -> BSPR_bBattUndrTempFault/1
  Bitwise Operator3/1 -> Compare To Constant5/1
  DFC_BoardTempTmt/1 -> Bitwise Operator3/1
  DFC_InCanBusOff/1 -> Bitwise Operator5/1
  Bitwise Operator5/1 -> Compare To Constant6/1
  Compare To Constant5/1 -> Logical Operator2/3
  Compare To Constant6/1 -> COMR_bCmuComBoff/1
  Bitwise Operator2/1 -> Compare To Constant4/1
  DFC_CellVoltTmt/1 -> Bitwise Operator2/1
  Compare To Constant4/1 -> Logical Operator2/2
  Bitwise Operator1/1 -> Compare To Constant3/1
  DFC_CellTempTmt/1 -> Bitwise Operator1/1
  Compare To Constant3/1 -> Logical Operator2/1
  Logical Operator2/1 -> COMR_bCmuComTOut/1
  DFC_DcCanBusOff/1 -> Bitwise Operator7/1
  Bitwise Operator7/1 -> Compare To Constant7/1
  Compare To Constant7/1 -> COMR_bDChrgComBoff/1
  DFC_VeCanBusOff/1 -> Bitwise Operator8/1
  Bitwise Operator8/1 -> Compare To Constant8/1
  Compare To Constant8/1 -> COMR_bEvComBoff/1
  Bitwise Operator9/1 -> Compare To Constant9/1
  Compare To Constant9/1 -> COMR_bVcuComTOut/1
  Bitwise Operator11/1 -> Compare To Constant11/1
  DFC_HvilMax/1 -> Bitwise Operator12/1
  Bitwise Operator12/1 -> Compare To Constant12/1
  Compare To Constant12/1 -> HVSR_bHvilInpScb/1
  DFC_HvilMin/1 -> Bitwise Operator13/1
  Bitwise Operator13/1 -> Compare To Constant13/1
  Compare To Constant13/1 -> HVSR_bHvilScg/1
  DFC_HvilSig/1 -> Bitwise Operator14/1
  Bitwise Operator14/1 -> Compare To Constant14/1
  Compare To Constant14/1 -> HVSR_bHvilOl/1
  DFC_CrashNpl/1 -> Bitwise Operator15/1
  Bitwise Operator15/1 -> Compare To Constant15/1
  Compare To Constant15/1 -> HVSR_bCrashFault/1
  DFC_Obc2E0Tmt/1 -> Bitwise Operator11/1

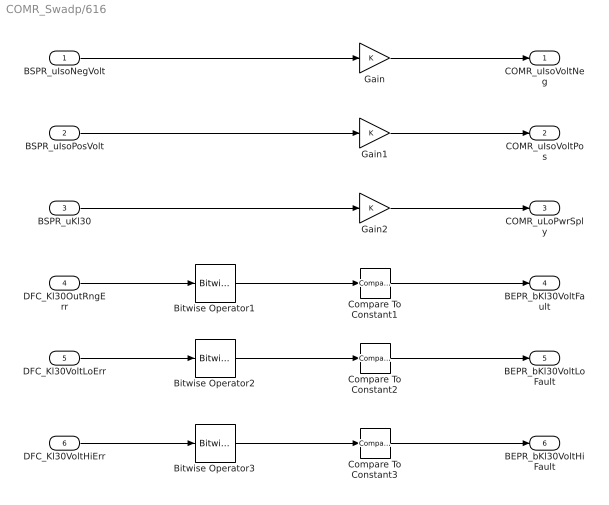
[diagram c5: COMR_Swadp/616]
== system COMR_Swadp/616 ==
  BSPR_uIsoNegVolt : Inport
  BSPR_uIsoPosVolt : Inport  Port=2
  BSPR_uKl30 : Inport  Port=3
  DFC_Kl30OutRngErr : Inport  Port=4
  DFC_Kl30VoltLoErr : Inport  Port=5
  DFC_Kl30VoltHiErr : Inport  Port=6
  Bitwise Operator1 : simulink/Logic and Bit Operations/Bitwise Operator  logicop=AND  UseBitMask=on  BitMask=bin2dec('00011000')  BitMaskRealWorld=Stored Integer
  Bitwise Operator2 : simulink/Logic and Bit Operations/Bitwise Operator  logicop=AND  UseBitMask=on  BitMask=bin2dec('00011000')  BitMaskRealWorld=Stored Integer
  Bitwise Operator3 : simulink/Logic and Bit Operations/Bitwise Operator  logicop=AND  UseBitMask=on  BitMask=bin2dec('00011000')  BitMaskRealWorld=Stored Integer
  Compare To Constant1 : simulink/Logic and Bit Operations/Compare To Constant  relop===  const=24  OutDataTypeStr=boolean
  Compare To Constant2 : simulink/Logic and Bit Operations/Compare To Constant  relop===  const=24  OutDataTypeStr=boolean
  Compare To Constant3 : simulink/Logic and Bit Operations/Compare To Constant  relop===  const=24  OutDataTypeStr=boolean
  Gain : Gain
  Gain1 : Gain
  Gain2 : Gain
  COMR_uIsoVoltNeg : Outport
  COMR_uIsoVoltPos : Outport  Port=2
  COMR_uLoPwrSply : Outport  Port=3
  BEPR_bKl30VoltFault : Outport  Port=4
  BEPR_bKl30VoltLoFault : Outport  Port=5
  BEPR_bKl30VoltHiFault : Outport  Port=6
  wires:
  BSPR_uIsoNegVolt/1 -> Gain/1
  BSPR_uIsoPosVolt/1 -> Gain1/1
  Gain/1 -> COMR_uIsoVoltNeg/1
  Gain1/1 -> COMR_uIsoVoltPos/1
  Gain2/1 -> COMR_uLoPwrSply/1
  BSPR_uKl30/1 -> Gain2/1
  DFC_Kl30OutRngErr/1 -> Bitwise Operator1/1
  DFC_Kl30VoltLoErr/1 -> Bitwise Operator2/1
  DFC_Kl30VoltHiErr/1 -> Bitwise Operator3/1
  Bitwise Operator1/1 -> Compare To Constant1/1
  Compare To Constant1/1 -> BEPR_bKl30VoltFault/1
  Bitwise Operator2/1 -> Compare To Constant2/1
  Compare To Constant2/1 -> BEPR_bKl30VoltLoFault/1
  Compare To Constant3/1 -> BEPR_bKl30VoltHiFault/1
  Bitwise Operator3/1 -> Compare To Constant3/1

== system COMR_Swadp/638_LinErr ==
  BSWLinCommunicationFault : Inport
  Constant1 : Constant  Value=COMR_ti638LinComErr_C
  Constant3 : Constant  Value=COMR_ti638LinComErr_C
  DSM_ReportCheck3 : Subsystem  TreatAsAtomicUnit=on  RTWFcnName=DSM_ReportCheck  RTWFileName=SrvLib
  Data Store Read : DataStoreRead  DataStoreName=DFC_638LinCommErr
  Data Store Write : DataStoreWrite  DataStoreName=DFC_638LinCommErr
  Logical Operator1 : Logic  Operator=NOT  AllPortsSameDT=off  OutDataTypeStr=boolean
  TONV_10msTimeDebounce1 : Subsystem  TreatAsAtomicUnit=on  RTWFcnName=TONV_10msTimeDebounce  RTWFileName=SrvLib
  TONV_10msTimeDebounce2 : Subsystem  TreatAsAtomicUnit=on  RTWFcnName=TONV_10msTimeDebounce  RTWFileName=SrvLib
  COMR_b638LinComErrDet : Outport
  COMR_b638LinComErrHeal : Outport  Port=2
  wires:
  Constant3/1 -> TONV_10msTimeDebounce2/2(T)
  BSWLinCommunicationFault/1 -> Logical Operator1/1, TONV_10msTimeDebounce2/1(u)
  TONV_10msTimeDebounce2/1(y) -> COMR_b638LinComErrDet/1, DSM_ReportCheck3/2(Err)
  Data Store Read/1 -> DSM_ReportCheck3/1(Dfc_id_nv)
  Logical Operator1/1 -> TONV_10msTimeDebounce1/1(u)
  Constant1/1 -> TONV_10msTimeDebounce1/2(T)
  TONV_10msTimeDebounce1/1(y) -> COMR_b638LinComErrHeal/1, DSM_ReportCheck3/3(Heal)
  DSM_ReportCheck3/1(Dfc_id) -> Data Store Write/1

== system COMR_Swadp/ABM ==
  DFC_ChkSumMsg050Err : Inport
  DFC_RcMsg050Mis : Inport  Port=2
  Bitwise Operator1 : simulink/Logic and Bit Operations/Bitwise Operator  logicop=AND  UseBitMask=on  BitMask=bin2dec('00011000')  BitMaskRealWorld=Stored Integer
  Bitwise Operator4 : simulink/Logic and Bit Operations/Bitwise Operator  logicop=AND  UseBitMask=on  BitMask=bin2dec('00011000')  BitMaskRealWorld=Stored Integer
  Compare To Constant1 : simulink/Logic and Bit Operations/Compare To Constant  relop===  const=24  OutDataTypeStr=boolean
  Compare To Constant2 : simulink/Logic and Bit Operations/Compare To Constant  relop===  const=24  OutDataTypeStr=boolean
  Logical Operator : Logic  Operator=NOR  AllPortsSameDT=off  OutDataTypeStr=boolean
  BSPR_flgGwAbmVld : Outport
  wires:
  Bitwise Operator1/1 -> Compare To Constant2/1
  Compare To Constant1/1 -> Logical Operator/1
  Logical Operator/1 -> BSPR_flgGwAbmVld/1
  Compare To Constant2/1 -> Logical Operator/2
  Bitwise Operator4/1 -> Compare To Constant1/1
  DFC_ChkSumMsg050Err/1 -> Bitwise Operator4/1
  DFC_RcMsg050Mis/1 -> Bitwise Operator1/1

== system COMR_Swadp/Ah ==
  Constant : Constant  Value=COMR_ahBattNrmCap_C
  COMR_ahCapacity : Outport
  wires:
  Constant/1 -> COMR_ahCapacity/1

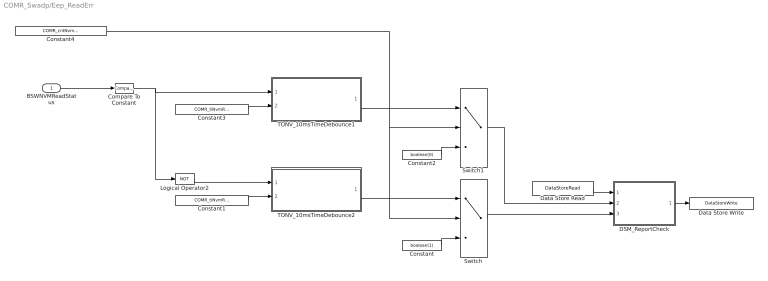
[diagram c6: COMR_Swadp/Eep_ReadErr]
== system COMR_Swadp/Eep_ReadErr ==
  BSWNVMReadStatus : Inport
  Compare To Constant : simulink/Logic and Bit Operations/Compare To Constant  relop===  const=1  OutDataTypeStr=boolean
  Constant : Constant  Value=boolean(1)  OutDataTypeStr=boolean
  Constant1 : Constant  Value=COMR_tiNvmReadErr_C
  Constant2 : Constant  Value=boolean(0)  OutDataTypeStr=boolean
  Constant3 : Constant  Value=COMR_tiNvmReadErr_C
  Constant4 : Constant  Value=COMR_cntNvmReadErr_CW
  DSM_ReportCheck : Subsystem  TreatAsAtomicUnit=on  RTWFcnName=DSM_ReportCheck  RTWFileName=SrvLib
  Data Store Read : DataStoreRead  DataStoreName=DFC_EepReadErr
  Data Store Write : DataStoreWrite  DataStoreName=DFC_EepReadErr
  Logical Operator2 : Logic  Operator=NOT  AllPortsSameDT=off  OutDataTypeStr=boolean
  Switch : Switch  Criteria=u2 > Threshold
  Switch1 : Switch  Criteria=u2 > Threshold
  TONV_10msTimeDebounce1 : Subsystem  TreatAsAtomicUnit=on  RTWFcnName=TONV_10msTimeDebounce  RTWFileName=SrvLib
  TONV_10msTimeDebounce2 : Subsystem  TreatAsAtomicUnit=on  RTWFcnName=TONV_10msTimeDebounce  RTWFileName=SrvLib
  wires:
  Compare To Constant/1 -> Logical Operator2/1, TONV_10msTimeDebounce1/1(u)
  Switch1/1 -> DSM_ReportCheck/2(Err)
  Constant3/1 -> TONV_10msTimeDebounce1/2(T)
  BSWNVMReadStatus/1 -> Compare To Constant/1
  Logical Operator2/1 -> TONV_10msTimeDebounce2/1(u)
  Constant1/1 -> TONV_10msTimeDebounce2/2(T)
  Switch/1 -> DSM_ReportCheck/3(Heal)
  DSM_ReportCheck/1(Dfc_id) -> Data Store Write/1
  Data Store Read/1 -> DSM_ReportCheck/1(Dfc_id_nv)
  TONV_10msTimeDebounce2/1(y) -> Switch/1
  TONV_10msTimeDebounce1/1(y) -> Switch1/1
  Constant/1 -> Switch/3
  Constant2/1 -> Switch1/3
  Constant4/1 -> Switch1/2, Switch/2

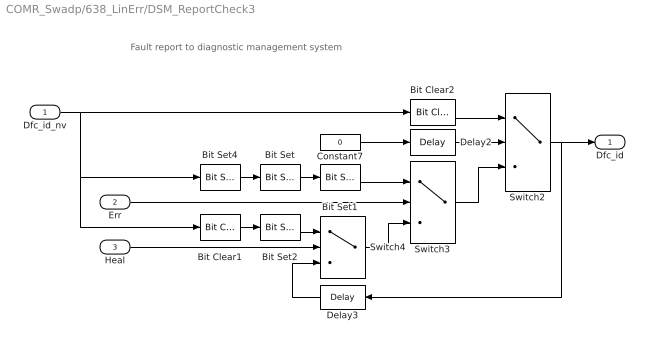
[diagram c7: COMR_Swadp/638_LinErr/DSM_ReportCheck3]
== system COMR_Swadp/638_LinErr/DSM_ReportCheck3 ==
  note: Fault report to diagnostic management system
  Dfc_id_nv : Inport  OutDataTypeStr=uint8
  Err : Inport  Port=2
  Heal : Inport  Port=3
  Bit Clear1 : simulink/Logic and Bit Operations/Bit Clear  iBit=4
  Bit Clear2 : simulink/Logic and Bit Operations/Bit Clear  iBit=3
  Bit Set : simulink/Logic and Bit Operations/Bit Set  iBit=4
  Bit Set1 : simulink/Logic and Bit Operations/Bit Set  iBit=3
  Bit Set2 : simulink/Logic and Bit Operations/Bit Set  iBit=3
  Bit Set4 : simulink/Logic and Bit Operations/Bit Set  iBit=7
  Constant7 : Constant  Value=0  OutDataTypeStr=boolean
  Delay2 : Delay  DelayLength=1  InitialCondition=1
  Delay3 : Delay  DelayLength=1  InitialCondition=0
  Switch2 : Switch  Criteria=u2 ~= 0
  Switch3 : Switch  Criteria=u2 ~= 0
  Switch4 : Switch  Criteria=u2 ~= 0
  Dfc_id : Outport  OutDataTypeStr=uint8
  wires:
  Dfc_id_nv/1 -> Bit Clear2/1, Bit Set4/1, Bit Clear1/1
  Bit Set4/1 -> Bit Set/1
  Constant7/1 -> Delay2/1
  Delay2/1 -> Switch2/2
  Switch3/1 -> Switch2/3
  Bit Clear2/1 -> Switch2/1
  Switch2/1 -> Delay3/1, Dfc_id/1
  Bit Set1/1 -> Switch3/1
  Bit Set/1 -> Bit Set1/1
  Switch4/1 -> Switch3/3
  Err/1 -> Switch3/2
  Bit Set2/1 -> Switch4/1
  Bit Clear1/1 -> Bit Set2/1
  Delay3/1 -> Switch4/3
  Heal/1 -> Switch4/2

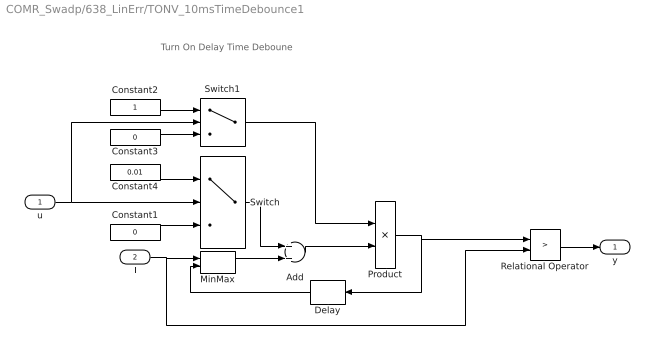
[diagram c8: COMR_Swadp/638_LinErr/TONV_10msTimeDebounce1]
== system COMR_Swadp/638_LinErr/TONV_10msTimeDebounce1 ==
  note: Turn On Delay Time Deboune
  u : Inport
  T : Inport  Port=2
  Add : Sum
  Constant1 : Constant  Value=0  OutDataTypeStr=single
  Constant2 : Constant  OutDataTypeStr=uint8
  Constant3 : Constant  Value=0  OutDataTypeStr=uint8
  Constant4 : Constant  Value=0.01  OutDataTypeStr=single
  Delay : Delay  DelayLength=1  InitialCondition=0
  MinMax : MinMax  Inputs=2
  Product : Product  OutMin=[0]  OutMax=[65535]  OutDataTypeStr=single
  Relational Operator : RelationalOperator  Operator=>  OutDataTypeStr=boolean  RndMeth=Simplest
  Switch : Switch  Criteria=u2 ~= 0
  Switch1 : Switch  Criteria=u2 ~= 0
  y : Outport
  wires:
  Switch1/1 -> Product/1
  Constant3/1 -> Switch1/3
  Constant2/1 -> Switch1/1
  u/1 -> Switch1/2, Switch/2
  Constant4/1 -> Switch/1
  Constant1/1 -> Switch/3
  Add/1 -> Product/2
  Product/1 -> Relational Operator/1, Delay/1
  Switch/1 -> Add/1
  Delay/1 -> MinMax/2
  Relational Operator/1 -> y/1
  T/1 -> MinMax/1, Relational Operator/2
  MinMax/1 -> Add/2

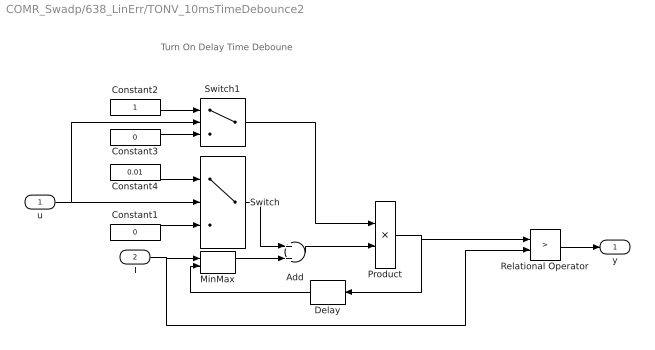
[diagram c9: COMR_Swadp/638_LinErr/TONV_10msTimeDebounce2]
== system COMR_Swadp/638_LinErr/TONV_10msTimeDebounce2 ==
  note: Turn On Delay Time Deboune
  u : Inport
  T : Inport  Port=2
  Add : Sum
  Constant1 : Constant  Value=0  OutDataTypeStr=single
  Constant2 : Constant  OutDataTypeStr=uint8
  Constant3 : Constant  Value=0  OutDataTypeStr=uint8
  Constant4 : Constant  Value=0.01  OutDataTypeStr=single
  Delay : Delay  DelayLength=1  InitialCondition=0
  MinMax : MinMax  Inputs=2
  Product : Product  OutMin=[0]  OutMax=[65535]  OutDataTypeStr=single
  Relational Operator : RelationalOperator  Operator=>  OutDataTypeStr=boolean  RndMeth=Simplest
  Switch : Switch  Criteria=u2 ~= 0
  Switch1 : Switch  Criteria=u2 ~= 0
  y : Outport
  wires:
  MinMax/1 -> Add/2
  T/1 -> Relational Operator/2, MinMax/1
  Relational Operator/1 -> y/1
  Delay/1 -> MinMax/2
  Switch/1 -> Add/1
  Product/1 -> Delay/1, Relational Operator/1
  Add/1 -> Product/2
  Constant1/1 -> Switch/3
  Constant4/1 -> Switch/1
  u/1 -> Switch/2, Switch1/2
  Constant2/1 -> Switch1/1
  Constant3/1 -> Switch1/3
  Switch1/1 -> Product/1

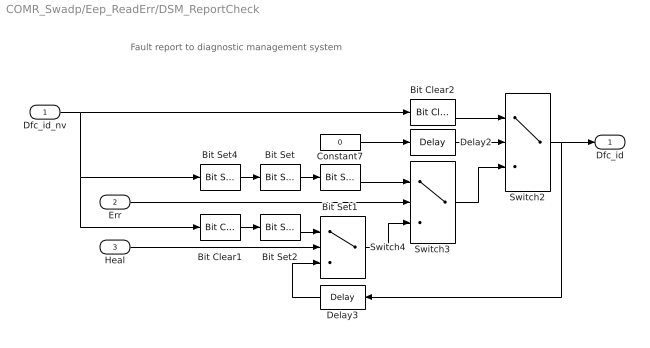
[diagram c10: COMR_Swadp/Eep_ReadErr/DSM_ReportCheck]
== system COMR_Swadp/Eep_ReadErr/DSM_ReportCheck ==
  note: Fault report to diagnostic management system
  Dfc_id_nv : Inport  OutDataTypeStr=uint8
  Err : Inport  Port=2
  Heal : Inport  Port=3
  Bit Clear1 : simulink/Logic and Bit Operations/Bit Clear  iBit=4
  Bit Clear2 : simulink/Logic and Bit Operations/Bit Clear  iBit=3
  Bit Set : simulink/Logic and Bit Operations/Bit Set  iBit=4
  Bit Set1 : simulink/Logic and Bit Operations/Bit Set  iBit=3
  Bit Set2 : simulink/Logic and Bit Operations/Bit Set  iBit=3
  Bit Set4 : simulink/Logic and Bit Operations/Bit Set  iBit=7
  Constant7 : Constant  Value=0  OutDataTypeStr=boolean
  Delay2 : Delay  DelayLength=1  InitialCondition=1
  Delay3 : Delay  DelayLength=1  InitialCondition=0
  Switch2 : Switch  Criteria=u2 ~= 0
  Switch3 : Switch  Criteria=u2 ~= 0
  Switch4 : Switch  Criteria=u2 ~= 0
  Dfc_id : Outport  OutDataTypeStr=uint8
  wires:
  Dfc_id_nv/1 -> Bit Clear2/1, Bit Set4/1, Bit Clear1/1
  Bit Set4/1 -> Bit Set/1
  Constant7/1 -> Delay2/1
  Delay2/1 -> Switch2/2
  Switch3/1 -> Switch2/3
  Bit Clear2/1 -> Switch2/1
  Switch2/1 -> Delay3/1, Dfc_id/1
  Bit Set1/1 -> Switch3/1
  Bit Set/1 -> Bit Set1/1
  Switch4/1 -> Switch3/3
  Err/1 -> Switch3/2
  Bit Set2/1 -> Switch4/1
  Bit Clear1/1 -> Bit Set2/1
  Delay3/1 -> Switch4/3
  Heal/1 -> Switch4/2

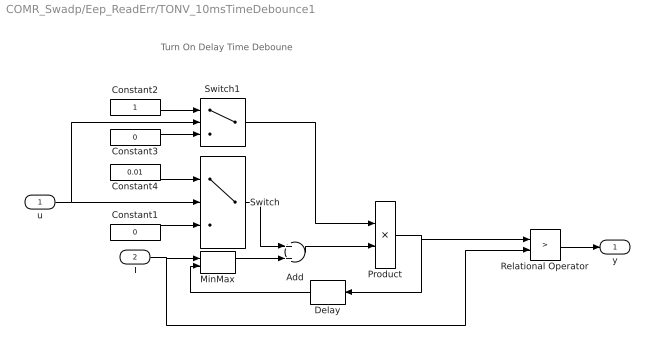
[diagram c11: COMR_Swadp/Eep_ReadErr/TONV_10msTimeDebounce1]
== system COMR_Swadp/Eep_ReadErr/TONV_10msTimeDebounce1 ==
  note: Turn On Delay Time Deboune
  u : Inport
  T : Inport  Port=2
  Add : Sum
  Constant1 : Constant  Value=0  OutDataTypeStr=single
  Constant2 : Constant  OutDataTypeStr=uint8
  Constant3 : Constant  Value=0  OutDataTypeStr=uint8
  Constant4 : Constant  Value=0.01  OutDataTypeStr=single
  Delay : Delay  DelayLength=1  InitialCondition=0
  MinMax : MinMax  Inputs=2
  Product : Product  OutMin=[0]  OutMax=[65535]  OutDataTypeStr=single
  Relational Operator : RelationalOperator  Operator=>  OutDataTypeStr=boolean  RndMeth=Simplest
  Switch : Switch  Criteria=u2 ~= 0
  Switch1 : Switch  Criteria=u2 ~= 0
  y : Outport
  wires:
  MinMax/1 -> Add/2
  T/1 -> Relational Operator/2, MinMax/1
  Relational Operator/1 -> y/1
  Delay/1 -> MinMax/2
  Switch/1 -> Add/1
  Product/1 -> Delay/1, Relational Operator/1
  Add/1 -> Product/2
  Constant1/1 -> Switch/3
  Constant4/1 -> Switch/1
  u/1 -> Switch/2, Switch1/2
  Constant2/1 -> Switch1/1
  Constant3/1 -> Switch1/3
  Switch1/1 -> Product/1

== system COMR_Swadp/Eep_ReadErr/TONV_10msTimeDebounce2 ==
  note: Turn On Delay Time Deboune
  u : Inport
  T : Inport  Port=2
  Add : Sum
  Constant1 : Constant  Value=0  OutDataTypeStr=single
  Constant2 : Constant  OutDataTypeStr=uint8
  Constant3 : Constant  Value=0  OutDataTypeStr=uint8
  Constant4 : Constant  Value=0.01  OutDataTypeStr=single
  Delay : Delay  DelayLength=1  InitialCondition=0
  MinMax : MinMax  Inputs=2
  Product : Product  OutMin=[0]  OutMax=[65535]  OutDataTypeStr=single
  Relational Operator : RelationalOperator  Operator=>  OutDataTypeStr=boolean  RndMeth=Simplest
  Switch : Switch  Criteria=u2 ~= 0
  Switch1 : Switch  Criteria=u2 ~= 0
  y : Outport
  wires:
  Switch1/1 -> Product/1
  Constant3/1 -> Switch1/3
  Constant2/1 -> Switch1/1
  u/1 -> Switch1/2, Switch/2
  Constant4/1 -> Switch/1
  Constant1/1 -> Switch/3
  Add/1 -> Product/2
  Product/1 -> Relational Operator/1, Delay/1
  Switch/1 -> Add/1
  Delay/1 -> MinMax/2
  Relational Operator/1 -> y/1
  T/1 -> MinMax/1, Relational Operator/2
  MinMax/1 -> Add/2

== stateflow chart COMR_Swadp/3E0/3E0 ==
  state Cell_Volt
    state CellVolt
      en:
      COMR_uCellVoltA = BSPR_uCellVolt_A[i];
      COMR_uCellVoltB = BSPR_uCellVolt_A[i+1];
      COMR_uCellVoltC = BSPR_uCellVolt_A[i+2];
      COMR_uCellVoltD = BSPR_uCellVolt_A[i+3];
      BSPR_cntCellSer = i/4;
    state CellVolt5
      en:
      i = i+4;
      COMR_uCellVoltA = BSPR_uCellVolt_A[i];
      COMR_uCellVoltB = 0;
      COMR_uCellVoltC = 0;
      COMR_uCellVoltD = 0;
      BSPR_cntCellSer = i/4;
    state CellVolt4
      en:
      i = i+4;
      COMR_uCellVoltA = BSPR_uCellVolt_A[i];
      COMR_uCellVoltB = BSPR_uCellVolt_A[i+1];
      COMR_uCellVoltC = 0;
      COMR_uCellVoltD = 0;
      BSPR_cntCellSer = i/4;
    state CellVolt3
      en:
      i = i+4;
      COMR_uCellVoltA = BSPR_uCellVolt_A[i];
      COMR_uCellVoltB = BSPR_uCellVolt_A[i+1];
      COMR_uCellVoltC = BSPR_uCellVolt_A[i+2];
      COMR_uCellVoltD = 0;
      BSPR_cntCellSer = i/4;
    (default) -> (junction 100)
    (junction 131) -> (junction 100)
    (junction 103) -> (junction 131)
    (junction 100) -> CellVolt : {i = 0;}
    (junction 101) -> CellVolt : {i = i + 4;}
    (junction 102) -> (junction 101)
    CellVolt -> (junction 102)
    CellVolt -> (junction 103) : [BSPR_cntCellSerNum - i == 4]
    (junction 130) -> (junction 103)
    CellVolt -> CellVolt5 : [ (BSPR_cntCellSerNum - i == 5)  ]
    CellVolt -> CellVolt4 : [ (BSPR_cntCellSerNum - i == 6)  ]
    CellVolt -> CellVolt3 : [(BSPR_cntCellSerNum - i == 7)  ]
    CellVolt5 -> (junction 104)
    CellVolt4 -> (junction 136)
    CellVolt3 -> (junction 121)
    (junction 104) -> (junction 130)
    (junction 136) -> (junction 104)
    (junction 121) -> (junction 136)
  data: BSPR_uCellVolt_A input single; i local uint8; BSPR_cntCellSer output uint8; COMR_uCellVoltA output single; COMR_uCellVoltB output single; COMR_uCellVoltC output single; COMR_uCellVoltD output single; BSPR_cntCellSerNum input
